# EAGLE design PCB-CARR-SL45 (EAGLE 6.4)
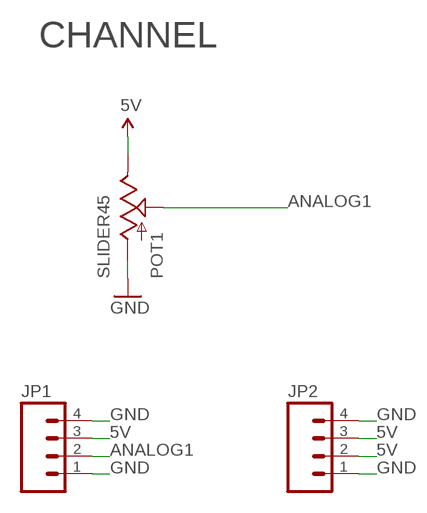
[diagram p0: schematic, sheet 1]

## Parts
JP1  M04PTH  [1X04]
JP2  M04PTH  [1X04]
POT1  SLIDER45  [SLIDER45]

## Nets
5V [Power]: JP1.3 JP2.2 JP2.3 POT1.1(E)
ANALOG1: JP1.2 POT1.2A(S)
GND [Power]: JP1.1 JP1.4 JP2.1 JP2.4 POT1.3(A)

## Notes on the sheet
- CHANNEL

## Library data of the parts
JP1 JP2 = SparkFun:M04: Header 4 Standard 4-pin 0.1" header. Use with straight break away headers (SKU : PRT-00116), right angle break away headers (PRT-00553), swiss pins (PRT-00743), machine pins (PRT-00117), and female headers (PRT-00115). Molex polarized connector foot print use with SKU : PRT-08231 with associated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
POT1 = SKAARHOJ:SLIDER

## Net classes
0 default: width 0.203 mm, drill 0.406 mm, clearance 0.152 mm
1 Power: width 0.406 mm, drill 0.61 mm, clearance 0.203 mm
2 Signal: width 0.152 mm, clearance 0.152 mm

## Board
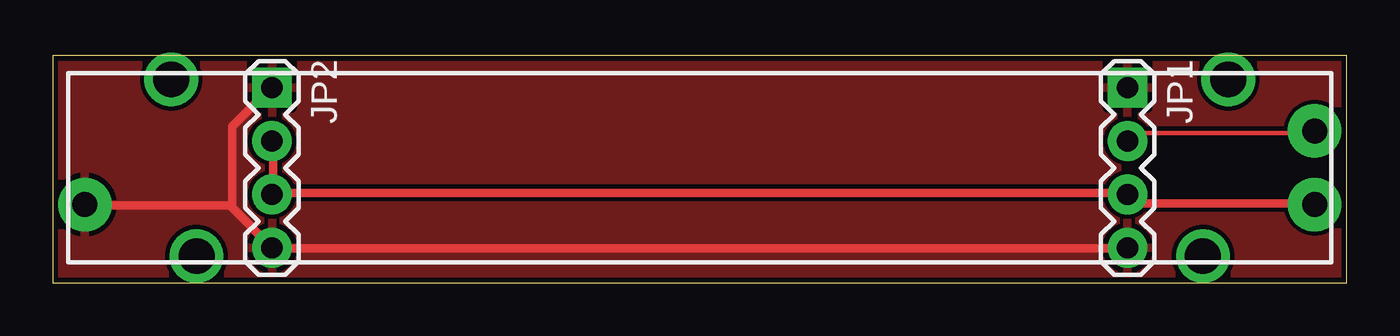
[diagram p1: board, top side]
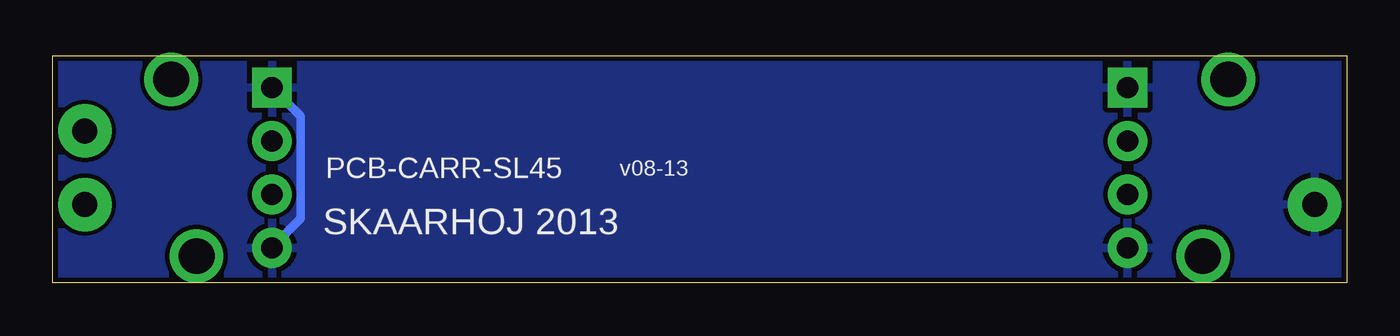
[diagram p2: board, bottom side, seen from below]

Size 61.47 x 10.79 mm. Coordinates in mm from the lower left corner, seen from the top.
Outline: 0,0 61.47,0 61.47,10.79 0,10.79 0,0
Copper layers (1*16): Top 0.035mm / dielectric 1.5mm / Bottom 0.035mm
Design rules "Fusion_eagle_rule_v1.1": minimum track width 6mil, minimum drill 12mil, track to track 6mil, track to pad 6mil, pad to pad 6mil, via to via 6mil, smd to smd 0mil, copper to edge 10mil, drill to drill 10mil, minimum pad ring 10mil, minimum via ring 6mil, stop-mask expansion 2mil, vias tented up to drill 100mil, thermal gap 10mil

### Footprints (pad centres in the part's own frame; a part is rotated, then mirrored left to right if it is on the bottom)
1X04 = drill 1.016 pad 1.88 square: 1 0,0 | drill 1.016 pad 1.88: 2 2.54,0; 3 5.08,0; 4 7.62,0
SLIDER45 = drill 1.194 pad 2.54: 1 -29.21,1.75; 2A -29.21,-1.75; 3 29.21,1.75 | drill 1.702: P$1 -23.9,4.2; P$2 23.9,4.2; P$3 25.1,-4.2; P$4 -25.1,-4.2

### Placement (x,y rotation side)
JP1  51.05,9.27 270 top
JP2  10.41,9.27 270 top
POT1  30.73,5.46 180 top

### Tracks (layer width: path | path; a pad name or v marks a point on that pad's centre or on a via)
5V
  Top 0.406: JP2.2 10.46,6.71 10.46,4.27 JP2.3 10.67,4.27 50.9,4.27 JP1.3 51.1,4.17 51.51,3.76 59.94,3.76 POT1.1
ANALOG1
  Top 0.203: JP1.2 51.1,6.81 51.41,7.11 59.94,7.11 POT1.2A
GND
  Top 0.406: 8.43,3.66 10.36,1.73 JP2.4 10.57,1.63 51,1.63 JP1.4 | 8.43,3.66 1.52,3.66 POT1.3 | JP2.1 10.36,9.25 8.53,7.42 8.53,3.76 8.43,3.66
  Bottom 0.406: JP1.4 51,1.73 49.68,3.05 49.68,7.92 51,9.25 JP1.1
  pour Top: 0,0 62.23,0 62.23,11.43 0,11.43
  pour Bottom: 0,0 62.23,0 62.23,11.43 0,11.43

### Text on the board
_bsilk: v08-13 | PCB-CARR-SL45 | SKAARHOJ 2013

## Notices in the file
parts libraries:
SparkFun: Licensing: CC v3.0 Share-Alike You are welcome to use this library for commercial purposes.
